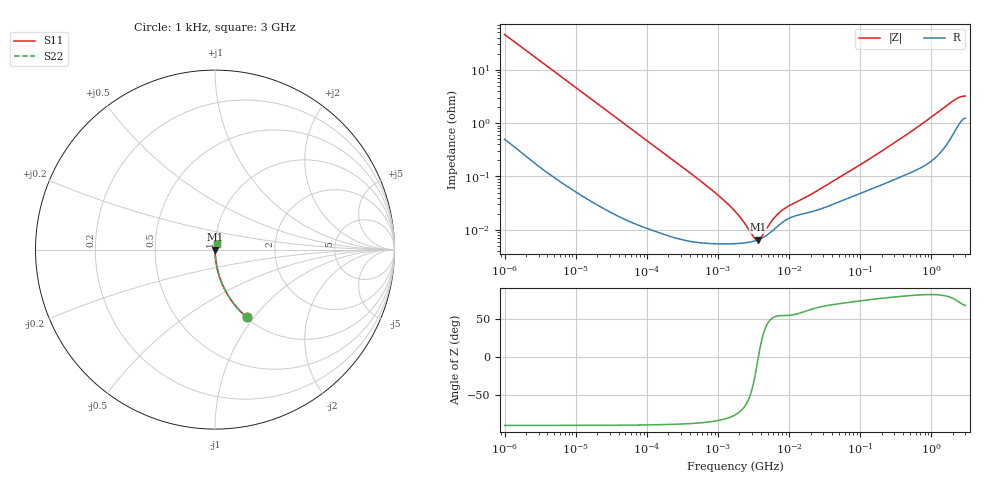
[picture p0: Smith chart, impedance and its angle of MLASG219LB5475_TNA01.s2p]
! MLASG219LB5475_TNA01  S-PARAMETER MODEL  ( Standard Model )
! Model Generated by TAIYO YUDEN Corporation (http://www.ty-top.com)
! Version 1.0
! TAIYO YUDEN Control No. 220601
! Copyright(c) 2015 TAIYO YUDEN CO.,LTD. All Rights Reserved.
! Product Description (link to TY-COMPAS)
! https://ds.yuden.co.jp/TYCOMPAS/or/detail?pn=MLASG219LB5475KTNA01&u=M
! Products Name : Multilayer Ceramic Capacitors
! Characteristics :
!  Capacitance : 4.7 [uF] , Rated Voltage : 35 [V] , TCC : X5R
!  Case Size : 2.0 x 1.25 / 0.079 x 0.049 [mm/inch] , Thickness : 0.85 / 0.033 [mm/inch]
!  (Conditions: Temperature = 25 [degC] , DC Bias Voltage = 0 [V])
! External Node Assignments :
!  1  o---| |---o  2
! GND o---------o GND
! Frequency Range : 1kHz  -  3GHz  [ 401 STEP ]
# MHZ S RI R 50
! Freq[MHz].  S11 Real  S11 Imag  S21 Real  S21 Imag  S12 Real  S12 Imag  S22 Real  S22 Imag
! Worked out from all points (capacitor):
!   401 points, 1 kHz to 3 GHz, reference 50 ohm
!   read as one part in series: C = 3.47 uF near 1.077 kHz
!   lowest |Z| = 6.52 mohm at 3.651 MHz (marker M1)
!   series resonance near 3.694 MHz, so ESL is about 530 pH
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0.001  0.1758 -0.3753  0.8242 0.3753  0.8242 0.3753  0.1758 -0.3753
0.001749  0.0668 -0.2444  0.9332 0.2444  0.9332 0.2444  0.0668 -0.2444
0.003297  0.0205 -0.1368  0.9795 0.1368  0.9795 0.1368  0.0205 -0.1368
0.005988  0.00673 -0.0767  0.9933 0.0767  0.9933 0.0767  0.00673 -0.0767
0.01216  0.00189 -0.0381  0.9981 0.0381  0.9981 0.0381  0.00189 -0.0381
0.147855  9.86e-05 -0.0032  0.9999 0.0032  0.9999 0.0032  9.86e-05 -0.0032
0.791611  5.56e-05 -0.000577  0.9999 0.000577  0.9999 0.000577  5.56e-05 -0.000577
1.238299  5.46e-05 -0.000344  0.9999 0.000344  0.9999 0.000344  5.46e-05 -0.000344
1.732051  5.51e-05 -0.000217  0.9999 0.000217  0.9999 0.000217  5.51e-05 -0.000217
2.709407  5.85e-05 -8.25e-05  0.9999 8.25e-05  0.9999 8.25e-05  5.85e-05 -8.25e-05
2.919173  5.96e-05 -6.23e-05  0.9999 6.23e-05  0.9999 6.23e-05  5.96e-05 -6.23e-05
3.651041  6.51e-05 -3.05e-06  0.9999 3.05e-06  0.9999 3.05e-06  6.51e-05 -3.05e-06
4.566395  7.56e-05 5.56e-05  0.9999 -5.56e-05  0.9999 -5.56e-05  7.56e-05 5.56e-05
4.919932  8.07e-05 7.51e-05  0.9999 -7.51e-05  0.9999 -7.51e-05  8.07e-05 7.51e-05
6.387174  0.000107 0.000141  0.9999 -0.000141  0.9999 -0.000141  0.000107 0.000141
7.988506  0.000137 0.000189  0.9999 -0.000189  0.9999 -0.000189  0.000137 0.000189
21.06097  0.00022 0.000421  0.9998 -0.000421  0.9998 -0.000421  0.00022 0.000421
256.0921  0.00081 0.00361  0.9992 -0.00361  0.9992 -0.00361  0.00081 0.00361
650.4536  0.00144 0.00847  0.9986 -0.00847  0.9986 -0.00847  0.00144 0.00847
2066.299  0.00715 0.0255  0.9929 -0.0255  0.9929 -0.0255  0.00715 0.0255
2489.759  0.0107 0.0284  0.9893 -0.0284  0.9893 -0.0284  0.0107 0.0284
3000  0.0131 0.0289  0.9869 -0.0289  0.9869 -0.0289  0.0131 0.0289
